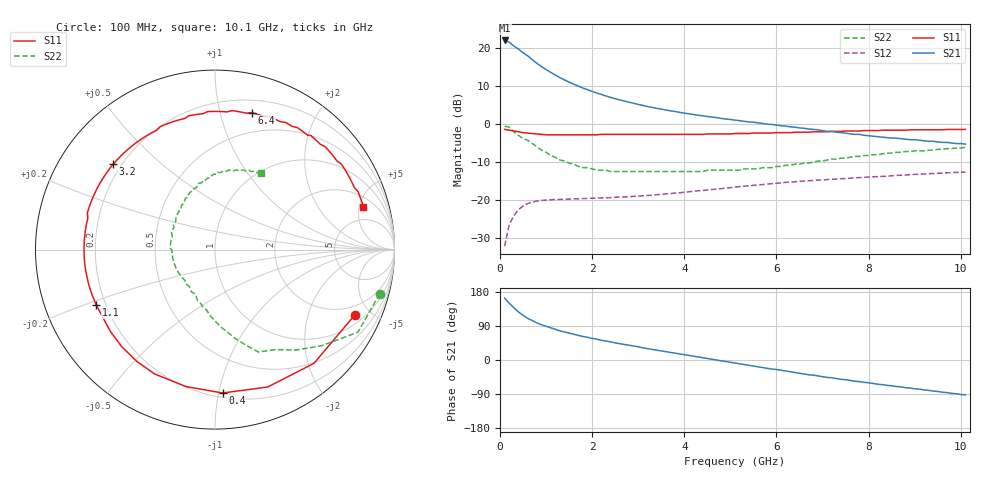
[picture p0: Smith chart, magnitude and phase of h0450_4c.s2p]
!HBFP-0450
!S and NOISE PARAMETERS at Vce=4V  Ic=5mA.  LAST UPDATED  09-04-98
# GHZ S MA R  50
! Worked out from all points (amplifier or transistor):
!   101 points, 100 MHz to 10.1 GHz, reference 50 ohm
!   highest |S21| = 22.1 dB at 100 MHz (marker M1)
!   |S21| within 3 dB of that: start of sweep to 477 MHz
!   unconditionally stable (mu >= 1): 2.985 GHz to end of sweep
!   at 1.7 GHz: K = 0.61, MSG = 14.8 dB, |S12| = -19.6 dB
!   at 5.1 GHz: K = 1.22, MAG = 6.0 dB, |S12| = -16.5 dB
!   at 10.1 GHz: K = 1.10, MAG = 1.8 dB, |S12| = -12.5 dB
!   lowest NFmin = 1.18 dB at 1.8 GHz
!   S11 on the Smith chart (normalised r, x): 100 MHz: 1.44, -4.02; 400 MHz: 0.23, -1.03; 1.1 GHz: 0.16, -0.22; 3.2 GHz: 0.17, +0.35; 6.4 GHz: 0.31, +1.26; 10.1 GHz: 3.02, +5.50
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0.1  0.86 -25.0  12.74 163.0  0.025 73.0  0.95 -15.0
0.2  0.84 -49.0  12.1 150.0  0.048 62.0  0.92 -30.0
0.3  0.82 -69.0  10.76 138.0  0.063 53.0  0.8 -42.0
0.4  0.8 -87.0  9.83 127.0  0.076 45.0  0.72 -51.0
0.5  0.78 -102.0  8.79 118.0  0.084 38.0  0.65 -59.0
0.6  0.77 -116.0  8 110.0  0.091 33.0  0.62 -67.0
0.7  0.76 -125.0  7.12 104.0  0.095 29.0  0.56 -72.0
0.8  0.75 -134.0  6.38 98.0  0.098 25.0  0.51 -77.0
0.9  0.74 -142.0  5.79 93.0  0.1 23.0  0.46 -82.0
1.1  0.73 -155.0  4.85 85.0  0.102 18.0  0.39 -91.0
1.3  0.73 -165.0  4.13 77.0  0.103 15.0  0.34 -98.0
1.5  0.73 -174.0  3.61 71.0  0.104 13.0  0.31 -105.0
1.8  0.73 176.0  3.01 62.0  0.106 11.0  0.27 -115.0
2.2  0.74 164.0  2.48 52.0  0.108 9.0  0.25 -128.0
2.5  0.74 156.0  2.18 45.0  0.11 8.0  0.24 -136.0
3.2  0.74 140.0  1.72 30.0  0.116 6.0  0.24 -154.0
3.5  0.74 134.0  1.59 24.0  0.12 5.0  0.24 -161.0
5.1  0.76 101.0  1.14 -8.0  0.15 -4.0  0.25 164.0
6.4  0.79 75.0  0.92 -33.0  0.176 -17.0  0.3 131.0
6.8  0.8 68.0  0.86 -40.0  0.183 -21.0  0.32 122.0
8.5  0.84 40.0  0.66 -68.0  0.211 -40.0  0.42 89.0
10.1  0.86 16.0  0.55 -92.0  0.236 -62.0  0.5 59.0
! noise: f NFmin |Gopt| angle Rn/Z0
1.8  1.18  0.51  165  0.05
2  1.27  0.52  172  0.05
2.5  1.46  0.57  -170  0.05
3.5  1.79  0.65  -143  0.15
4  2.07  0.67  -130  0.27
5  2.46  0.72  -107  0.68
5.5  2.65  0.74  -95  1.03
7  3.21  0.78  -65  2.54
8  3.6  0.83  -47  3.92
10  4.34  0.84  -16  6.74
